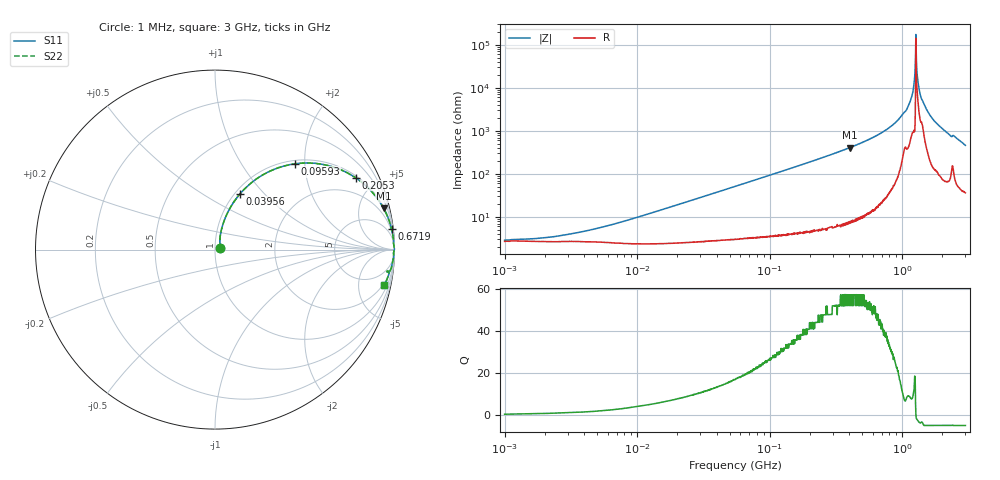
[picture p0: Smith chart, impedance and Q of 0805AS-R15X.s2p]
!s-Parameter Generated by FASTRON Sdn. Bhd.
!FASTRON P/N : 0805AS-R15X
!Keysight Technologies: E4991B_MY54100416_A.01.15
!Date: Mon Jun 15 12:52:31 2026
!Version  :Rev01  Mon Jun 15 12:52:31 2026
!Data & Calibration Information:
!Freq  S11  S21  S12  S22
!PortZ  Port1:50+j0  Port2:50+j0
!When reading reference impedance value at option line is always used.
! Remarks : This data is being provided solely for informational purposes.
# Hz S dB R 50
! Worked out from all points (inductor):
!   1601 points, 1 MHz to 3 GHz, reference 50 ohm
!   read as one part in series: L = 151 nH near 7.742 MHz
!   highest Q = 57.3 at 403.3 MHz (marker M1), where L = 161 nH
!   self-resonance near 1.269 GHz
!   S11 on the Smith chart (normalised r, x): 1 MHz: 1.05, +0.02; 39.56 MHz: 1.06, +0.74; 95.93 MHz: 1.07, +1.78; 205.3 MHz: 1.09, +3.86; 671.9 MHz: 1, +17; 3 GHz: 1.73, -9.19
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1000000  -31.10 19.0  -0.23 -0.5  -0.23 -0.5  -31.10 19.0
3804036  -27.20 51.8  -0.23 -2.0  -0.23 -2.0  -27.20 51.8
1.447069e7  -17.40 72.5  -0.28 -7.6  -0.28 -7.6  -17.40 72.5
3.956422e7  -9.39 65.9  -0.77 -19.8  -0.77 -19.8  -9.39 65.9
5.504702e7  -7.01 60.2  -1.22 -26.4  -1.22 -26.4  -7.01 60.2
9.593103e7  -3.70 47.0  -2.70 -40.7  -2.70 -40.7  -3.70 47.0
2.052512e8  -1.11 27.1  -6.84 -61.6  -6.84 -61.6  -1.11 27.1
2.083556e8  -1.08 26.7  -6.95 -61.9  -6.95 -61.9  -1.08 26.7
4.033367e8  -0.29 13.7  -12.50 -75.3  -12.50 -75.3  -0.29 13.7
6.719458e8  -0.08 6.8  -18.60 -81.9  -18.60 -81.9  -0.08 6.8
7.925923e8  -0.05 4.9  -21.40 -83.4  -21.40 -83.4  -0.05 4.9
9.349007e8  -0.04 3.1  -25.20 -84.0  -25.20 -84.0  -0.04 3.1
1.10276e9  -0.03 1.6  -31.00 -82.1  -31.00 -82.1  -0.03 1.6
1.182785e9  -0.02 0.9  -36.10 -81.7  -36.10 -81.7  -0.02 0.9
1.237271e9  -0.00 0.4  -43.60 -86.0  -43.60 -86.0  -0.00 0.4
1.274982e9  -0.01 -0.1  -58.30 50.9  -58.30 50.9  -0.01 -0.1
1.307284e9  -0.02 -0.3  -44.30 68.2  -44.30 68.2  -0.02 -0.3
1.347129e9  -0.03 -0.6  -38.90 73.7  -38.90 73.7  -0.03 -0.6
1.395152e9  -0.04 -1.0  -35.00 72.8  -35.00 72.8  -0.04 -1.0
1.629261e9  -0.04 -2.5  -27.10 82.7  -27.10 82.7  -0.04 -2.5
2.255531e9  -0.15 -6.8  -18.50 78.5  -18.50 78.5  -0.15 -6.8
3e9  -0.34 -12.0  -13.60 73.5  -13.60 73.5  -0.34 -12.0
